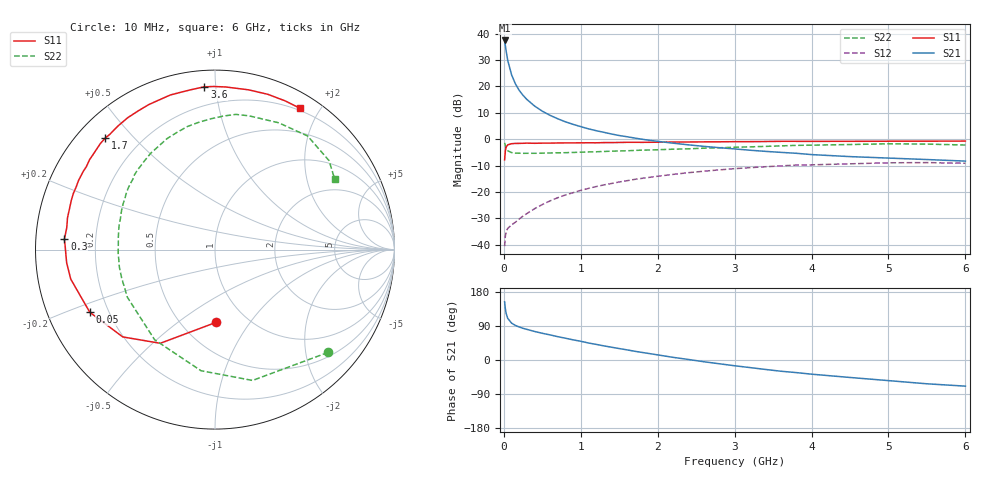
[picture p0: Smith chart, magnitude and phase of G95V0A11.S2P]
! SIEMENS Small Signal Semiconductors
! BFG235
! Si NPN RF Bipolar Junction Transistor in SOT223
! VCE = 5 V  IC = 110 mA
! Common Emitter S-Parameters:  July  1994
# GHz  S  MA  R  50
!  f  S11  S21  S12  S22
! GHz  MAG  ANG  MAG  ANG  MAG  ANG  MAG  ANG
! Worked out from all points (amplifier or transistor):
!   40 points, 10 MHz to 6 GHz, reference 50 ohm
!   highest |S21| = 37.4 dB at 10 MHz (marker M1)
!   |S21| within 3 dB of that: start of sweep to 25.06 MHz
!   unconditionally stable (mu >= 1): 464.3 MHz to 1.449 GHz
!   at 200 MHz: K = 0.78, MSG = 24.4 dB, |S12| = -30.3 dB
!   at 1.5 GHz: K = 0.99, MSG = 8.8 dB, |S12| = -16.2 dB
!   at 6 GHz: K = 0.89, MSG = 0.4 dB, |S12| = -9.1 dB
!   S11 on the Smith chart (normalised r, x): 10 MHz: 0.73, -0.70; 50 MHz: 0.13, -0.23; 300 MHz: 0.09, +0.03; 1.7 GHz: 0.08, +0.42; 3.6 GHz: 0.09, +0.93; 6 GHz: 0.17, +1.76
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0.01  0.4051 -89.0  73.97 153.5  0.0094 65.9  0.8513 -42.3
0.02  0.6047 -120.3  58.9 134.9  0.0148 49.1  0.7584 -74.0
0.03  0.7078 -136.6  46.69 122.9  0.0174 42.0  0.6792 -96.6
0.05  0.78 -153.4  31.33 110.0  0.0204 33.8  0.6045 -123.8
0.1  0.8202 -168.4  16.63 97.4  0.0237 35.7  0.5558 -151.4
0.15  0.8298 -174.9  11.18 91.2  0.0267 41.1  0.5436 -163.1
0.2  0.8314 -178.3  8.379 87.1  0.0307 45.4  0.5418 -169.5
0.25  0.8351 178.6  6.746 83.6  0.0349 49.2  0.5389 -174.0
0.3  0.8411 176.1  5.635 80.8  0.039 52.6  0.5396 -177.7
0.4  0.8349 171.5  4.235 75.3  0.0482 55.4  0.5394 177.1
0.5  0.8407 167.8  3.383 70.5  0.0577 56.7  0.5428 172.8
0.6  0.8417 164.7  2.827 66.3  0.0676 57.1  0.547 169.0
0.8  0.849 158.4  2.131 57.5  0.0877 55.8  0.5538 162.3
1.1  0.8536 149.3  1.567 44.9  0.1167 51.4  0.5723 153.3
1.4  0.8611 142.2  1.251 33.7  0.1448 45.8  0.5916 145.1
1.7  0.8715 134.6  1.05 23.1  0.1729 39.6  0.6118 137.3
2.2  0.8812 123.4  0.839 7.0  0.215 28.6  0.6452 123.7
3.2  0.8973 102.0  0.617 -20.0  0.2883 5.4  0.7143 97.6
3.6  0.9089 93.7  0.562 -29.6  0.3114 -4.5  0.7455 86.4
4.5  0.9096 78.2  0.467 -46.1  0.3409 -24.4  0.7907 63.3
5.5  0.9161 64.8  0.411 -62.8  0.3597 -46.4  0.8059 38.0
6  0.9188 58.9  0.384 -69.0  0.3494 -54.8  0.774 30.5
